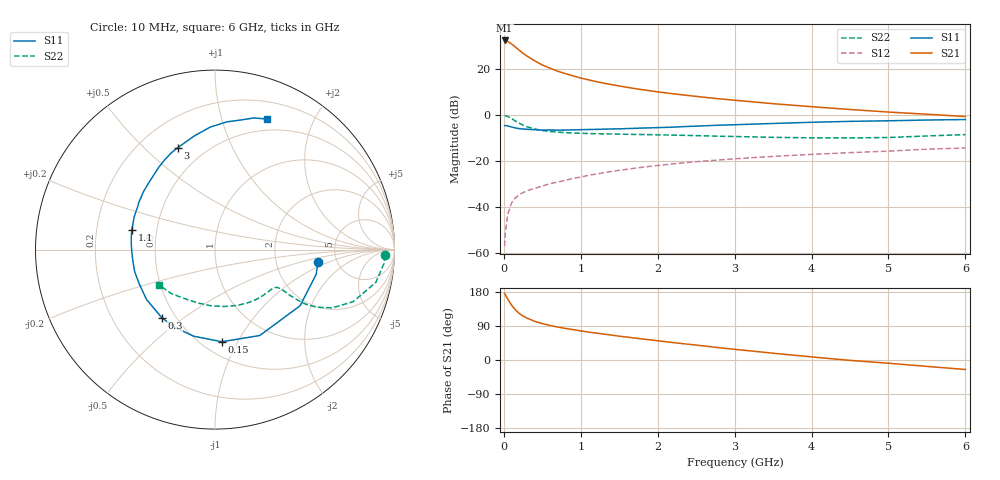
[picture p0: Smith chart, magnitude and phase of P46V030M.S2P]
! SIEMENS Small Signal Semiconductors
! BFP182
! Si NPN RF Bipolar Junction Transistor in SOT143
! VCE = 6 V  IC = 30 mA
! Common Emitter S-Parameters:  March  1996
# GHz  S  MA  R  50
!  f  S11  S21  S12  S22
! GHz  MAG  ANG  MAG  ANG  MAG  ANG  MAG  ANG
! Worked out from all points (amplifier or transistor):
!   36 points, 10 MHz to 6 GHz, reference 50 ohm
!   highest |S21| = 32.2 dB at 10 MHz (marker M1)
!   |S21| within 3 dB of that: start of sweep to 155.6 MHz
!   unconditionally stable (mu >= 1): 651.8 MHz to 5.449 GHz
!   at 250 MHz: K = 0.57, MSG = 30.2 dB, |S12| = -33.8 dB
!   at 1.4 GHz: K = 1.19, MAG = 16.2 dB, |S12| = -24.7 dB
!   at 6 GHz: K = 0.96, MSG = 6.8 dB, |S12| = -14.4 dB
!   S11 on the Smith chart (normalised r, x): 10 MHz: 3.58, -0.72; 150 MHz: 0.62, -0.86; 300 MHz: 0.42, -0.42; 1.1 GHz: 0.36, +0.10; 3 GHz: 0.36, +0.64; 6 GHz: 0.37, +1.41
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0.01  0.5777 -6.7  40.75 175.6  0.0014 75.5  0.947 -1.9
0.02  0.5804 -13.7  40.65 172.2  0.0028 77.8  0.9458 -4.5
0.05  0.5681 -33.4  39.18 160.9  0.0069 80.1  0.9144 -11.5
0.1  0.5398 -62.5  34.21 144.9  0.0121 64.1  0.8223 -20.7
0.15  0.5147 -85.8  29.37 132.5  0.0156 59.0  0.7299 -26.4
0.2  0.4969 -103.8  25.06 123.0  0.0185 55.4  0.6523 -29.5
0.25  0.4876 -117.6  21.46 116.0  0.0204 53.6  0.5919 -31.0
0.3  0.4816 -128.0  18.76 110.8  0.0223 52.6  0.5469 -31.4
0.4  0.472 -144.1  14.75 102.1  0.0252 52.7  0.4884 -31.4
0.5  0.4633 -156.2  12 96.1  0.0283 52.5  0.4533 -31.0
0.6  0.4642 -164.9  10.21 91.1  0.0318 54.4  0.4315 -30.8
0.7  0.4619 -171.8  8.763 87.0  0.0344 55.3  0.4173 -31.0
0.8  0.4635 -178.1  7.775 83.3  0.0376 55.8  0.4073 -31.3
1  0.4725 171.1  6.235 76.8  0.0442 56.4  0.3938 -32.6
1.1  0.4762 166.5  5.703 73.7  0.0482 56.4  0.3894 -33.7
1.5  0.4911 151.8  4.189 62.8  0.0619 55.4  0.378 -38.7
2.2  0.5359 130.0  2.84 46.0  0.0855 50.7  0.3601 -50.6
3  0.6042 110.2  2.056 28.2  0.1103 43.5  0.3358 -67.6
3.5  0.6435 100.4  1.73 17.9  0.124 39.1  0.3218 -80.0
4.5  0.7152 84.6  1.294 -1.0  0.15 30.4  0.3123 -107.5
5.5  0.7651 73.5  1.021 -16.9  0.1781 22.2  0.3451 -134.6
6  0.7836 68.1  0.912 -25.0  0.1896 17.2  0.3689 -147.5
